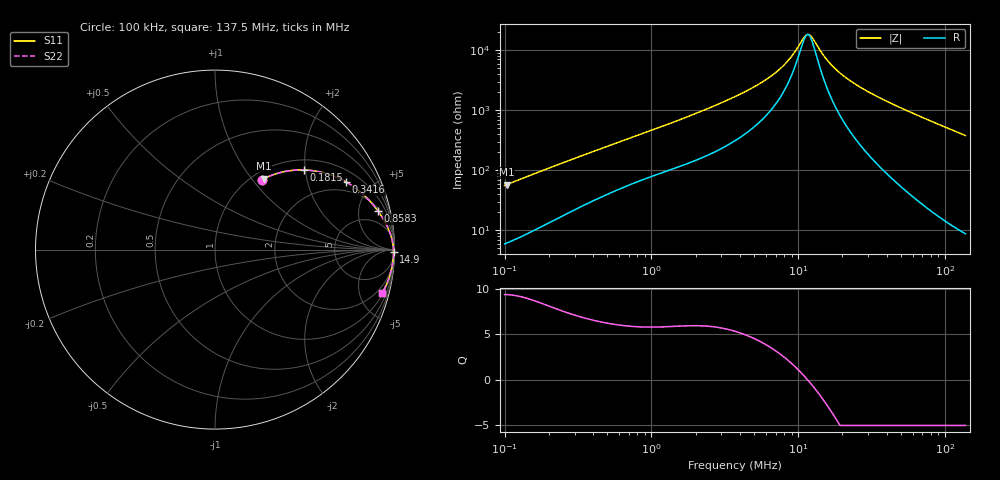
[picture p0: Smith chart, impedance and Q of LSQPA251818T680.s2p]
! LSQPA251818T680  S-PARAMETER MODEL  ( General Type )
! Model Generated by TAIYO YUDEN Corporation (http://www.ty-top.com)
! Version 3.0
! TAIYO YUDEN Control No. 160907NF25SB-FAC
! Copyright(c) 2007 TAIYO YUDEN CO.,LTD. All Rights Reserved.
! Product Description (link to TY-COMPAS)
! https://ds.yuden.co.jp/TYCOMPAS/or/detail?pn=LSQPA251818T680K&u=M
! Products Name : Inductors
! Characteristics :
!  Inductance : 68 uH , SRF(min) : 9.5 MHz , DC Resistance(max) : 3.64 Ohm
!  Rated Current : Saturation :200 mA , Temp Rise : 200 mA (40 degC)
!  Case Size : 2.5 x 1.8 / 0.098 x 0.071 [mm/inch] , Thickness : 1.8 / 0.071 [mm/inch]
!  (Conditions: Temperature = 25 degC , DC Bias Current/Voltage = 0A / 0V)
! External Node Assignments :
!  1  o---GGG---o  2
! GND o---------o GND
! Frequency Range : 0.1MHz  -  137.487582MHz  [ 402 STEP ]
# MHz S RI R 50
! Freq[MHz].  S11 Real  S11 Imag  S21 Real  S21 Imag  S12 Real  S12 Imag  S22 Real  S22 Imag
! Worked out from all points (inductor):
!   401 points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, 100 kHz to 137.5 MHz, reference 50 ohm
!   read as one part in series: L = 87.8 uH near 103.7 kHz
!   highest Q = 9.35 at 103.7 kHz (marker M1), where L = 88.5 uH
!   self-resonance near 11.57 MHz
!   S11 on the Smith chart (normalised r, x): 100 kHz: 1.12, +1.11; 181.5 kHz: 1.24, +1.97; 341.6 kHz: 1.51, +3.52; 858.3 kHz: 2.37, +7.96; 14.9 MHz: open; 137.5 MHz: 1.18, -7.58
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0.1  0.2601 0.3885  0.7399 -0.3885  0.7399 -0.3885  0.2601 0.3885
0.103679  0.2724 0.3949  0.7276 -0.3949  0.7276 -0.3949  0.2724 0.3949
0.181513  0.4963 0.4437  0.5037 -0.4437  0.5037 -0.4437  0.4963 0.4437
0.335474  0.7257 0.3793  0.2743 -0.3793  0.2743 -0.3793  0.7257 0.3793
0.34159  0.7312 0.3762  0.2688 -0.3762  0.2688 -0.3762  0.7312 0.3762
0.526988  0.8372 0.2969  0.1628 -0.2969  0.1628 -0.2969  0.8372 0.2969
0.858289  0.9098 0.213  0.0902 -0.213  0.0902 -0.213  0.9098 0.213
1.125429  0.9359 0.1735  0.0641 -0.1735  0.0641 -0.1735  0.9359 0.1735
3.707932  0.9859 0.0569  0.0141 -0.0569  0.0141 -0.0569  0.9859 0.0569
5.226359  0.9902 0.0368  0.00982 -0.0368  0.00982 -0.0368  0.9902 0.0368
6.730363  0.9922 0.0242  0.00778 -0.0242  0.00778 -0.0242  0.9922 0.0242
8.667178  0.9936 0.0126  0.00639 -0.0126  0.00639 -0.0126  0.9936 0.0126
11.16136  0.9945 0.00162  0.00553 -0.00162  0.00553 -0.00162  0.9945 0.00162
11.78295  0.9946 -0.000734  0.00541 0.000734  0.00541 0.000734  0.9946 -0.000734
12.43915  0.9947 -0.0031  0.0053 0.0031  0.0053 0.0031  0.9947 -0.0031
14.9021  0.9949 -0.0111  0.00511 0.0111  0.00511 0.0111  0.9949 -0.0111
17.53309  0.9949 -0.0187  0.00512 0.0187  0.00512 0.0187  0.9949 -0.0187
21.77741  0.9945 -0.0297  0.00546 0.0297  0.00546 0.0297  0.9945 -0.0297
29.07615  0.9934 -0.0466  0.00662 0.0466  0.00662 0.0466  0.9934 -0.0466
41.73016  0.9902 -0.0733  0.00983 0.0733  0.00983 0.0733  0.9902 -0.0733
77.12628  0.9748 -0.1413  0.0252 0.1413  0.0252 0.1413  0.9748 -0.1413
137.4876  0.93 -0.2439  0.07 0.2439  0.07 0.2439  0.93 -0.2439
